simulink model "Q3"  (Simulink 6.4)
settings: Solver=ode4  StartTime=0.0  StopTime=10  FixedStep=0.01  RelTol=1e-3
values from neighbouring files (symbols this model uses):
  A = pi*R^2    (= 0.0669661890039)    [par.m]
  a = 14    [par.m]
  Cd = 0.02    [par.m]
  Cd_sfe = 0.24    [par.m]
  g = 9.81    [par.m]
  h = -0.012    [par.m]
  I = diag([Ix Iy Iz])    [par.m]
  I_inv = inv(I)    [par.m]
  J = Ja+Jr/(n^2)    (= 2.07047193878e-06)    [par.m]
  Ja = 1e-006    (= 1e-06)    [par.m]
  Jr = 3.357e-005    (= 3.357e-05)    [par.m]
  K = 0.00345    [par.m]
  l = 0.237    [par.m]
  m = 0.488    [par.m]
  Minv = inv(M)    [par.m]
  n = 5.6    [par.m]
  omegah = x    (= 300)    [par.m]
  r = 0.1    [par.m]
  R = 0.146    [par.m]
  rho = 1.225    [par.m]
  s = b*c*R/A    (= 0.100289416195)    [par.m]
  tau = Ra*J/K^2    (= 0.22300735354)    [par.m]
  teta = 0.22    [par.m]
  x0 = []    [betaDx.m]    (also in alfa.m; control.m = zeros(16,1); beta.m; lambda.m)
libraries: aerolibutil x11, simulink x8, aerosimlib x8
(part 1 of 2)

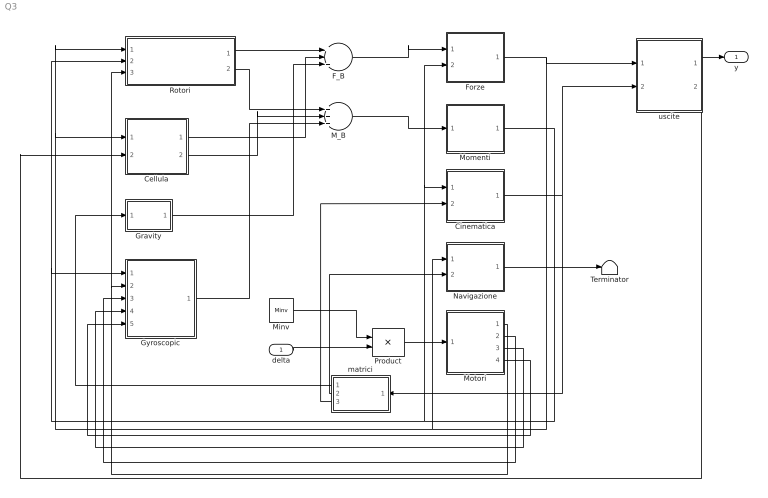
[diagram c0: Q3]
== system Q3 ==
  delta : Inport
  Cellula : Subsystem
  Cinematica : Subsystem
  F_B : Sum  Inputs=+++  OutScaling=2^-10
  Forze : Subsystem
  Gravity : Subsystem
  Gyroscopic : Subsystem
  M_B : Sum  Inputs=+++  OutScaling=2^-10
  Minv : Constant  Value=Minv  OutDataType=sfix(16)  ConRadixGroup=Use specified scaling  OutScaling=2^0  SampleTime=inf  FramePeriod=inf
  Momenti : Subsystem
  Motori : Subsystem
  Navigazione : Subsystem
  Product : Product  Multiplication=Matrix(*)
  Rotori : Subsystem
  Terminator : Terminator
  matrici : Subsystem  Orientation=left
  uscite : Subsystem
  y : Outport
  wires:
  Rotori/1(F_R) -> F_B/1
  Cellula/1(F_C) -> F_B/2
  Rotori/2(M_R) -> M_B/1
  Cellula/2(M_C) -> M_B/2
  F_B/1 -> Forze/1(F_B)
  M_B/1 -> Momenti/1(M_B)
  Cinematica/1(Euler) -> matrici/1(Euler), uscite/2(Euler)
  matrici/3(R_inv) -> Cinematica/2(R_inv)
  Momenti/1(omegaB) -> Gyroscopic/1(omegaB), Rotori/2(omegaB), Cinematica/1(omegaB), Forze/2(omegaB)
  Forze/1(velB) -> Cellula/1(velB), Rotori/1(velB), Navigazione/1(velB), uscite/1(velB)
  Motori/1(omega_r) -> Gyroscopic/2(omega_r), Rotori/3(omega_r)
  Product/1 -> Motori/1(Va)
  Motori/2(omega_m) -> Gyroscopic/3(omega_m)
  Motori/3(omega_r_dot) -> Gyroscopic/4(omega_r_dot)
  Motori/4(omega_m_dot) -> Gyroscopic/5(omega_m_dot)
  matrici/1(L_BE) -> Gravity/1(L_BE)
  matrici/2(L_EB) -> Navigazione/2(L_EB)
  uscite/1(y) -> y/1
  Navigazione/1(NED) -> Terminator/1
  uscite/2(ab) -> Cellula/2(ab)
  Minv/1 -> Product/1
  delta/1 -> Product/2
  Gyroscopic/1(M_G) -> M_B/3
  Gravity/1(F_g) -> F_B/3

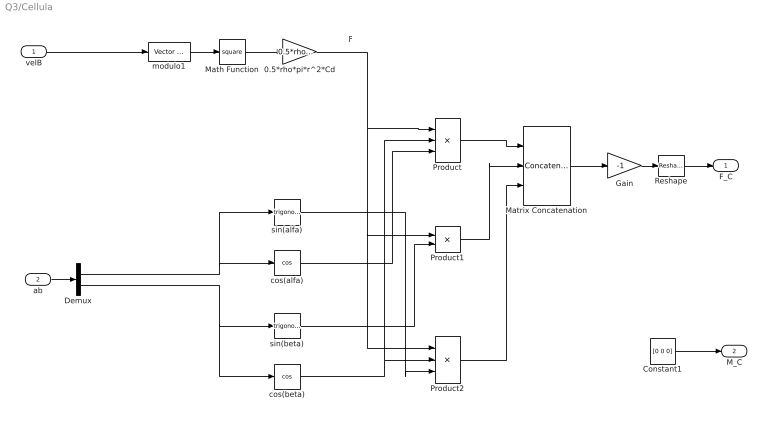
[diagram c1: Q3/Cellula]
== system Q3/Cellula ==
  note: F
  velB : Inport
  ab : Inport  Port=2
  0.5*rho*pi*r^2*Cd : Gain  Gain=0.5*rho*pi*r^2*Cd_sfe
  Constant1 : Constant  Value=[0 0 0]  OutDataType=sfix(16)  ConRadixGroup=Use specified scaling  OutScaling=2^0  SampleTime=inf  FramePeriod=inf
  Demux : Demux  Outputs=2
  Gain : Gain  Gain=-1
  Math Function : Math  Operator=square
  Matrix Concatenation : Concatenate  NumInputs=3  Mode=Vertical matrix concatenation
  Product : Product  Inputs=3
  Product1 : Product
  Product2 : Product  Inputs=3
  Reshape : simulink/Math Operations/Reshape  OutputDimensionality=1-D array  OutputDimensions=[1,1]
  cos(alfa) : Trigonometry  Operator=cos
  cos(beta) : Trigonometry  Operator=cos
  modulo1 : aerosimlib/Math/Vector norm  SystemSampleTime=-1
  sin(alfa) : Trigonometry
  sin(beta) : Trigonometry
  F_C : Outport
  M_C : Outport  Port=2
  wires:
  modulo1/1 -> Math Function/1
  Math Function/1 -> 0.5*rho*pi*r^2*Cd/1
  Constant1/1 -> M_C/1
  ab/1 -> Demux/1
  Demux/1 -> cos(alfa)/1, sin(alfa)/1
  Demux/2 -> sin(beta)/1, cos(beta)/1
  0.5*rho*pi*r^2*Cd/1 -> Product/1, Product1/1, Product2/1
  cos(beta)/1 -> Product/2, Product2/2
  cos(alfa)/1 -> Product/3
  sin(beta)/1 -> Product1/2
  sin(alfa)/1 -> Product2/3
  Product/1 -> Matrix Concatenation/1
  Product1/1 -> Matrix Concatenation/2
  Product2/1 -> Matrix Concatenation/3
  Matrix Concatenation/1 -> Gain/1
  Gain/1 -> Reshape/1
  Reshape/1 -> F_C/1
  velB/1 -> modulo1/1

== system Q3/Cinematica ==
  note: [p q r]
  note: Euler_dot
  note: [phi teta psi]
  omegaB : Inport
  R_inv : Inport  Port=2
  Integrator : Integrator  InitialCondition=[x0(4) x0(5) x0(6)]
  Product : Product  Multiplication=Matrix(*)
  Euler : Outport
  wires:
  R_inv/1 -> Product/1
  omegaB/1 -> Product/2
  Product/1 -> Integrator/1
  Integrator/1 -> Euler/1

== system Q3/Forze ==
  note: [X Y Z]
  note: acc
  note: vel_dot
  note: [u v w]
  F_B : Inport
  omegaB : Inport  Port=2
  Divide : Product  Inputs=*/  OutScaling=2^-10
  Gain : Gain  Gain=-1
  Integrator : Integrator  InitialCondition=[x0(1) x0(2) x0(3)]
  Sum : Sum  Inputs=++|
  massa : Constant  Value=m  OutDataType=sfix(16)  ConRadixGroup=Use specified scaling  OutScaling=2^0  SampleTime=inf  FramePeriod=inf
  omegaB x vel : aerolibutil/3x3 Cross Product  SystemSampleTime=-1
  velB : Outport
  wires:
  omegaB/1 -> omegaB x vel/1
  omegaB x vel/1 -> Gain/1
  F_B/1 -> Divide/1
  massa/1 -> Divide/2
  Divide/1 -> Sum/1
  Gain/1 -> Sum/2
  Sum/1 -> Integrator/1
  Integrator/1 -> velB/1, omegaB x vel/2

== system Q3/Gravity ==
  L_BE : Inport
  Constant : Constant  Value=[0 0 m*g]'  OutDataType=sfix(16)  ConRadixGroup=Use specified scaling  OutScaling=2^0  SampleTime=inf  FramePeriod=inf
  L_BE1 : Product  Multiplication=Matrix(*)
  F_g : Outport
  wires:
  Constant/1 -> L_BE1/2
  L_BE1/1 -> F_g/1
  L_BE/1 -> L_BE1/1

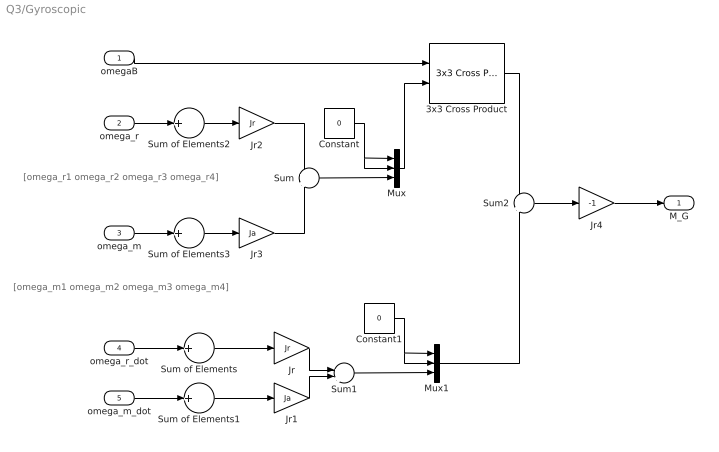
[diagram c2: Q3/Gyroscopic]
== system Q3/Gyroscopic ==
  note: [omega_r1 omega_r2 omega_r3 omega_r4]
  note: [omega_m1 omega_m2 omega_m3 omega_m4]
  omegaB : Inport
  omega_r : Inport  Port=2
  omega_m : Inport  Port=3
  omega_r_dot : Inport  Port=4
  omega_m_dot : Inport  Port=5
  3x3 Cross Product : aerolibutil/3x3 Cross Product  SystemSampleTime=-1
  Constant : Constant  Value=0  OutDataType=sfix(16)  ConRadixGroup=Use specified scaling  OutScaling=2^0  SampleTime=inf  FramePeriod=inf
  Constant1 : Constant  Value=0  OutDataType=sfix(16)  ConRadixGroup=Use specified scaling  OutScaling=2^0  SampleTime=inf  FramePeriod=inf
  Jr : Gain  Gain=Jr
  Jr1 : Gain  Gain=Ja
  Jr2 : Gain  Gain=Jr
  Jr3 : Gain  Gain=Ja
  Jr4 : Gain  Gain=-1
  Mux : Mux  Inputs=3
  Mux1 : Mux  Inputs=3
  Sum : Sum  Inputs=+|+
  Sum of Elements{,1..3} (4 alike) : Sum  Inputs=+  OutScaling=2^-10
  Sum1 : Sum  Inputs=+|+
  Sum2 : Sum  Inputs=+|+
  M_G : Outport
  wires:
  omega_r_dot/1 -> Sum of Elements/1
  omega_m_dot/1 -> Sum of Elements1/1
  Sum of Elements/1 -> Jr/1
  Sum of Elements1/1 -> Jr1/1
  omegaB/1 -> 3x3 Cross Product/1
  omega_r/1 -> Sum of Elements2/1
  omega_m/1 -> Sum of Elements3/1
  Sum of Elements2/1 -> Jr2/1
  Sum of Elements3/1 -> Jr3/1
  Jr2/1 -> Sum/1
  Jr3/1 -> Sum/2
  Jr/1 -> Sum1/1
  Jr1/1 -> Sum1/2
  Sum2/1 -> Jr4/1
  Jr4/1 -> M_G/1
  Sum/1 -> Mux/3
  Constant/1 -> Mux/1, Mux/2
  Mux/1 -> 3x3 Cross Product/2
  3x3 Cross Product/1 -> Sum2/1
  Sum1/1 -> Mux1/3
  Constant1/1 -> Mux1/1, Mux1/2
  Mux1/1 -> Sum2/2

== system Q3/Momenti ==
  note: [l m n]
  note: omegaB_dot
  M_B : Inport
  Gain : Gain  Gain=-1
  I * omegaB : Product  Multiplication=Matrix(*)
  I*omegaB2 : Product  Multiplication=Matrix(*)
  Integrator : Integrator  InitialCondition=[x0(7) x0(8) x0(9)]
  Scope3 : Scope
  Sum : Sum  Inputs=|++
  matrice d'inerzia  inversa in assi corpo : Constant  Value=I_inv  OutDataType=sfix(16)  ConRadixGroup=Use specified scaling  OutScaling=2^0  SampleTime=inf  FramePeriod=inf
  matrice d'inerzia in assi corpo : Constant  Value=I  OutDataType=sfix(16)  ConRadixGroup=Use specified scaling  OutScaling=2^0  SampleTime=inf  FramePeriod=inf
  omegaB x (I * omegaB) : aerolibutil/3x3 Cross Product  SystemSampleTime=-1
  omegaB : Outport
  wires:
  matrice d'inerzia in assi corpo/1 -> I * omegaB/1
  I * omegaB/1 -> omegaB x (I * omegaB)/2
  omegaB x (I * omegaB)/1 -> Gain/1
  Gain/1 -> Sum/1
  M_B/1 -> Sum/2
  Integrator/1 -> omegaB/1, I * omegaB/2, omegaB x (I * omegaB)/1
  matrice d'inerzia  inversa in assi corpo/1 -> I*omegaB2/1
  Sum/1 -> I*omegaB2/2
  I*omegaB2/1 -> Integrator/1, Scope3/1

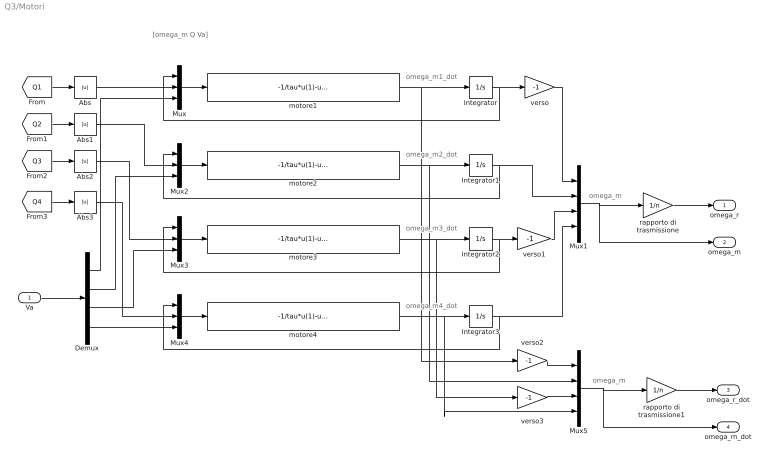
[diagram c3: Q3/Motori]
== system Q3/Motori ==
  note: [omega_m Q Va]
  note: omega_m1_dot
  note: omega_m2_dot
  note: omega_m3_dot
  note: omega_m4_dot
  note: omega_m
  note: omega_m
  Va : Inport
  Abs{,1..3} (4 alike) : Abs  SampleTime=-1
  Demux : Demux
  Integrator : Integrator  InitialCondition=x0(10)
  Integrator1 : Integrator  InitialCondition=x0(11)
  Integrator2 : Integrator  InitialCondition=x0(12)
  Integrator3 : Integrator  InitialCondition=x0(13)
  Mux{,2..4} (4 alike) : Mux  Inputs=3
  Mux1 : Mux
  Mux5 : Mux
  motore{1..4} (4 alike) : Fcn  Expr=-1/tau*u(1)-u(2)/J/n+1/K/tau*u(3)
  rapporto di trasmissione : Gain  Gain=1/n
  rapporto di trasmissione1 : Gain  Gain=1/n
  verso{,1..3} (4 alike) : Gain  Gain=-1
  omega_r : Outport
  omega_m : Outport  Port=2
  omega_r_dot : Outport  Port=3
  omega_m_dot : Outport  Port=4
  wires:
  Mux/1 -> motore1/1
  motore1/1 -> Integrator/1, verso2/1
  Integrator/1 -> Mux/1, verso/1
  Mux1/1 -> rapporto di trasmissione/1, omega_m/1
  Va/1 -> Demux/1
  Demux/1 -> Mux/3
  Mux2/1 -> motore2/1
  motore2/1 -> Integrator1/1, Mux5/2
  Integrator1/1 -> Mux2/1, Mux1/2
  Mux3/1 -> motore3/1
  motore3/1 -> Integrator2/1, verso3/1
  Integrator2/1 -> Mux3/1, verso1/1
  Mux4/1 -> motore4/1
  motore4/1 -> Integrator3/1, Mux5/4
  Integrator3/1 -> Mux4/1, Mux1/4
  Demux/2 -> Mux2/3
  Demux/3 -> Mux3/3
  Demux/4 -> Mux4/3
  [Q1] -> Abs/1
  [Q2] -> Abs1/1
  [Q3] -> Abs2/1
  [Q4] -> Abs3/1
  rapporto di trasmissione/1 -> omega_r/1
  Mux5/1 -> omega_m_dot/1, rapporto di trasmissione1/1
  rapporto di trasmissione1/1 -> omega_r_dot/1
  Abs/1 -> Mux/2
  Abs1/1 -> Mux2/2
  Abs2/1 -> Mux3/2
  Abs3/1 -> Mux4/2
  verso3/1 -> Mux5/3
  verso2/1 -> Mux5/1
  verso1/1 -> Mux1/3
  verso/1 -> Mux1/1

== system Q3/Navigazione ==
  note: [u v w]
  note: NED_dot
  note: [N E D]
  velB : Inport
  L_EB : Inport  Port=2
  Integrator : Integrator  InitialCondition=[x0(14) x0(15) x0(16)]
  Product : Product  Multiplication=Matrix(*)
  NED : Outport
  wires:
  velB/1 -> Product/2
  Product/1 -> Integrator/1
  Integrator/1 -> NED/1
  L_EB/1 -> Product/1

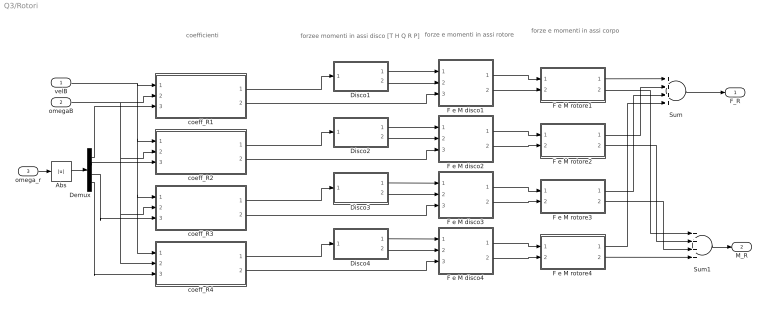
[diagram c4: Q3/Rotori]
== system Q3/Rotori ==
  note: coefficienti
  note: forzee momenti in assi disco [T H Q R P]
  note: forze e momenti in assi rotore
  note: forze e momenti in assi corpo
  velB : Inport
  omegaB : Inport  Port=2
  omega_r : Inport  Port=3
  Abs : Abs  SampleTime=-1
  Demux : Demux
  Disco1 : Subsystem
  Disco2 : Subsystem
  Disco3 : Subsystem
  Disco4 : Subsystem
  F e M disco1 : Subsystem
  F e M disco2 : Subsystem
  F e M disco3 : Subsystem
  F e M disco4 : Subsystem
  F e M rotore1 : Subsystem
  F e M rotore2 : Subsystem
  F e M rotore3 : Subsystem
  F e M rotore4 : Subsystem
  Sum : Sum  Inputs=++++
  Sum1 : Sum  Inputs=++++
  coeff_R1 : Subsystem
  coeff_R2 : Subsystem
  coeff_R3 : Subsystem
  coeff_R4 : Subsystem
  F_R : Outport
  M_R : Outport  Port=2
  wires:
  F e M disco1/1(F_disco1) -> F e M rotore1/1(F_disco1)
  F e M disco1/2(M_disco1) -> F e M rotore1/2(M_disco1)
  F e M disco2/1(F_disco2) -> F e M rotore2/1(F_disco2)
  F e M disco2/2(M_disco2) -> F e M rotore2/2(M_disco2)
  F e M disco3/1(F_disco3) -> F e M rotore3/1(F_disco3)
  F e M disco3/2(M_disco3) -> F e M rotore3/2(M_disco3)
  F e M disco4/1(F_disco4) -> F e M rotore4/1(F_disco4)
  F e M disco4/2(M_disco4) -> F e M rotore4/2(M_disco4)
  Disco1/1(F_D1) -> F e M disco1/1(F_D1)
  Disco1/2(M_D1) -> F e M disco1/2(M_D1)
  Disco2/1(F_D2) -> F e M disco2/1(F_D2)
  Disco2/2(M_D2) -> F e M disco2/2(M_D2)
  Disco3/1(F_D3) -> F e M disco3/1(F_D3)
  Disco3/2(M_D3) -> F e M disco3/2(M_D3)
  Disco4/1(F_D4) -> F e M disco4/1(F_D4)
  Disco4/2(M_D4) -> F e M disco4/2(M_D4)
  coeff_R4/1(coeff4) -> Disco4/1(coeff4)
  coeff_R3/1(coeff3) -> Disco3/1(coeff3)
  coeff_R2/1(coeff2) -> Disco2/1(coeff2)
  coeff_R1/1(coeff1) -> Disco1/1(coeff1)
  coeff_R1/2(L_RD1) -> F e M disco1/3(L_RD1)
  coeff_R2/2(L_RD2) -> F e M disco2/3(L_RD2)
  coeff_R3/2(L_RD3) -> F e M disco3/3(L_RD3)
  coeff_R4/2(L_RD4) -> F e M disco4/3(L_RD4)
  velB/1 -> coeff_R4/1(velB), coeff_R3/1(velB), coeff_R2/1(velB), coeff_R1/1(velB)
  omegaB/1 -> coeff_R3/2(omegaB), coeff_R4/2(omegaB), coeff_R2/2(omegaB), coeff_R1/2(omegaB)
  F e M rotore1/1(F_R1) -> Sum/1
  F e M rotore2/1(F_R2) -> Sum/2
  F e M rotore3/1(F_R3) -> Sum/3
  F e M rotore4/1(F_R4) -> Sum/4
  Sum/1 -> F_R/1
  F e M rotore1/2(M_R1) -> Sum1/1
  F e M rotore2/2(M_R2) -> Sum1/2
  F e M rotore3/2(M_R3) -> Sum1/3
  F e M rotore4/2(M_R4) -> Sum1/4
  Sum1/1 -> M_R/1
  omega_r/1 -> Abs/1
  Demux/1 -> coeff_R1/3(omega_r1)
  Demux/2 -> coeff_R2/3(omega_r2)
  Demux/3 -> coeff_R3/3(omega_r3)
  Demux/4 -> coeff_R4/3(omega_r4)
  Abs/1 -> Demux/1

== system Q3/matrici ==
  Euler : Inport
  Subsystem1 : Subsystem
  Subsystem2 : Subsystem
  hlpfcn : Subsystem
  L_BE : Outport
  L_EB : Outport  Port=2
  R_inv : Outport  Port=3
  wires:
  hlpfcn/1(hlpfcn) -> Subsystem1/1(hlpfcn), Subsystem2/1(hlpfcn)
  Subsystem1/1(L_BE) -> L_BE/1
  Euler/1 -> hlpfcn/1(Euler)
  Subsystem2/1(R_inv) -> R_inv/1
  Subsystem1/2(L_EB) -> L_EB/1

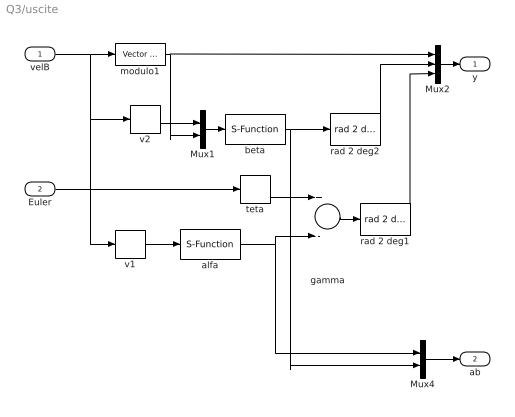
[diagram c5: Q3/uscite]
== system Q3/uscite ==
  velB : Inport
  Euler : Inport  Port=2
  Mux1 : Mux  Inputs=2
  Mux2 : Mux  Inputs=3
  Mux4 : Mux  Inputs=2
  alfa : S-Function  FunctionName=alfa
  beta : S-Function  FunctionName=beta
  gamma : Sum  Inputs=+-  OutScaling=2^-10
  modulo1 : aerosimlib/Math/Vector norm  SystemSampleTime=-1
  rad 2 deg1 : aerosimlib/Unit Conversion/Angular position/rad 2 deg  SystemSampleTime=-1
  rad 2 deg2 : aerosimlib/Unit Conversion/Angular position/rad 2 deg  SystemSampleTime=-1
  teta : Selector  Elements=2  InputPortWidth=3
  v1 : Selector  Elements=[1 3]  InputPortWidth=3
  v2 : Selector  Elements=2  InputPortWidth=3
  y : Outport
  ab : Outport  Port=2
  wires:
  modulo1/1 -> Mux1/2, Mux2/1
  Mux1/1 -> beta/1
  v2/1 -> Mux1/1
  beta/1 -> rad 2 deg2/1, Mux4/2
  rad 2 deg2/1 -> Mux2/2
  Mux2/1 -> y/1
  teta/1 -> gamma/1
  gamma/1 -> rad 2 deg1/1
  alfa/1 -> gamma/2, Mux4/1
  v1/1 -> alfa/1
  rad 2 deg1/1 -> Mux2/3
  Euler/1 -> teta/1
  velB/1 -> modulo1/1, v2/1, v1/1
  Mux4/1 -> ab/1

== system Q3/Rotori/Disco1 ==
  coeff1 : Inport
  Constant : Constant  Value=0  OutDataType=sfix(16)  ConRadixGroup=Use specified scaling  OutScaling=2^0  SampleTime=inf  FramePeriod=inf
  H : Fcn  Expr=-rho*s*A*u(1)^2*R^2*u(3)
  Mux : Mux  Inputs=3
  Mux1 : Mux  Inputs=3
  Mux2 : Mux  Inputs=[1 5]
  P : Fcn  Expr=rho*s*A*u(1)^2*R^3*u(6)
  Q : Fcn  Expr=rho*s*A*u(1)^2*R^3*u(4)
  R : Fcn  Expr=-rho*s*A*u(1)^2*R^3*u(5)
  T : Fcn  Expr=-rho*s*A*u(1)^2*R^2*u(2)
  omegah : Constant  Value=omegah  OutDataType=sfix(16)  ConRadixGroup=Use specified scaling  OutScaling=2^0  SampleTime=inf  FramePeriod=inf
  F_D1 : Outport
  M_D1 : Outport  Port=2
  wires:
  Constant/1 -> Mux/2
  H/1 -> Mux/1
  T/1 -> Mux/3
  R/1 -> Mux1/1
  Q/1 -> Mux1/3, [Q1]
  Mux/1 -> F_D1/1
  Mux1/1 -> M_D1/1
  Mux2/1 -> T/1, Q/1, R/1, P/1, H/1
  omegah/1 -> Mux2/1
  coeff1/1 -> Mux2/2
  P/1 -> Mux1/2

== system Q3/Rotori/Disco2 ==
  coeff2 : Inport
  Constant : Constant  Value=0  OutDataType=sfix(16)  ConRadixGroup=Use specified scaling  OutScaling=2^0  SampleTime=inf  FramePeriod=inf
  H : Fcn  Expr=-rho*s*A*u(1)^2*R^2*u(3)
  Mux : Mux  Inputs=3
  Mux1 : Mux  Inputs=3
  Mux2 : Mux  Inputs=[1 5]
  P : Fcn  Expr=rho*s*A*u(1)^2*R^3*u(6)
  Q : Fcn  Expr=-rho*s*A*u(1)^2*R^3*u(4)
  R : Fcn  Expr=rho*s*A*u(1)^2*R^3*u(5)
  T : Fcn  Expr=-rho*s*A*u(1)^2*R^2*u(2)
  omegah : Constant  Value=omegah  OutDataType=sfix(16)  ConRadixGroup=Use specified scaling  OutScaling=2^0  SampleTime=inf  FramePeriod=inf
  F_D2 : Outport
  M_D2 : Outport  Port=2
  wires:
  Constant/1 -> Mux/2
  H/1 -> Mux/1
  T/1 -> Mux/3
  R/1 -> Mux1/1
  Q/1 -> Mux1/3, [Q2]
  Mux/1 -> F_D2/1
  Mux1/1 -> M_D2/1
  Mux2/1 -> T/1, Q/1, R/1, P/1, H/1
  omegah/1 -> Mux2/1
  coeff2/1 -> Mux2/2
  P/1 -> Mux1/2

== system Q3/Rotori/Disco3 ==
  coeff3 : Inport
  Constant : Constant  Value=0  OutDataType=sfix(16)  ConRadixGroup=Use specified scaling  OutScaling=2^0  SampleTime=inf  FramePeriod=inf
  H : Fcn  Expr=-rho*s*A*u(1)^2*R^2*u(3)
  Mux : Mux  Inputs=3
  Mux1 : Mux  Inputs=3
  Mux2 : Mux  Inputs=[1 5]
  P : Fcn  Expr=rho*s*A*u(1)^2*R^3*u(6)
  Q : Fcn  Expr=rho*s*A*u(1)^2*R^3*u(4)
  R : Fcn  Expr=-rho*s*A*u(1)^2*R^3*u(5)
  T : Fcn  Expr=-rho*s*A*u(1)^2*R^2*u(2)
  omegah : Constant  Value=omegah  OutDataType=sfix(16)  ConRadixGroup=Use specified scaling  OutScaling=2^0  SampleTime=inf  FramePeriod=inf
  F_D3 : Outport
  M_D3 : Outport  Port=2
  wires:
  Constant/1 -> Mux/2
  H/1 -> Mux/1
  T/1 -> Mux/3
  R/1 -> Mux1/1
  Q/1 -> Mux1/3, [Q3]
  Mux/1 -> F_D3/1
  Mux1/1 -> M_D3/1
  Mux2/1 -> T/1, Q/1, R/1, P/1, H/1
  omegah/1 -> Mux2/1
  coeff3/1 -> Mux2/2
  P/1 -> Mux1/2

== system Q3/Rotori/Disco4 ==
  coeff4 : Inport
  Constant : Constant  Value=0  OutDataType=sfix(16)  ConRadixGroup=Use specified scaling  OutScaling=2^0  SampleTime=inf  FramePeriod=inf
  H : Fcn  Expr=-rho*s*A*u(1)^2*R^2*u(3)
  Mux : Mux  Inputs=3
  Mux1 : Mux  Inputs=3
  Mux2 : Mux  Inputs=[1 5]
  P : Fcn  Expr=rho*s*A*u(1)^2*R^3*u(6)
  Q : Fcn  Expr=-rho*s*A*u(1)^2*R^3*u(4)
  R : Fcn  Expr=rho*s*A*u(1)^2*R^3*u(5)
  T : Fcn  Expr=-rho*s*A*u(1)^2*R^2*u(2)
  omegah : Constant  Value=omegah  OutDataType=sfix(16)  ConRadixGroup=Use specified scaling  OutScaling=2^0  SampleTime=inf  FramePeriod=inf
  F_D4 : Outport
  M_D4 : Outport  Port=2
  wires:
  Constant/1 -> Mux/2
  H/1 -> Mux/1
  T/1 -> Mux/3
  R/1 -> Mux1/1
  Q/1 -> Mux1/3, [Q4]
  Mux/1 -> F_D4/1
  Mux1/1 -> M_D4/1
  Mux2/1 -> T/1, Q/1, R/1, P/1, H/1
  omegah/1 -> Mux2/1
  coeff4/1 -> Mux2/2
  P/1 -> Mux1/2

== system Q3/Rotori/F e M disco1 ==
  note: in assi disco
  F_D1 : Inport
  M_D1 : Inport  Port=2
  L_RD1 : Inport  Port=3
  L_RD x F_D : Product  Multiplication=Matrix(*)
  Product1 : Product  Multiplication=Matrix(*)
  F_disco1 : Outport
  M_disco1 : Outport  Port=2
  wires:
  F_D1/1 -> L_RD x F_D/2
  M_D1/1 -> Product1/2
  L_RD x F_D/1 -> F_disco1/1
  Product1/1 -> M_disco1/1
  L_RD1/1 -> L_RD x F_D/1, Product1/1

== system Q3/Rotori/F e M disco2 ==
  note: in assi disco
  F_D2 : Inport
  M_D2 : Inport  Port=2
  L_RD2 : Inport  Port=3
  L_RD x F_D : Product  Multiplication=Matrix(*)
  Product1 : Product  Multiplication=Matrix(*)
  F_disco2 : Outport
  M_disco2 : Outport  Port=2
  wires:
  F_D2/1 -> L_RD x F_D/2
  M_D2/1 -> Product1/2
  L_RD x F_D/1 -> F_disco2/1
  Product1/1 -> M_disco2/1
  L_RD2/1 -> L_RD x F_D/1, Product1/1

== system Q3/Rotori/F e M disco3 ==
  note: in assi disco
  F_D3 : Inport
  M_D3 : Inport  Port=2
  L_RD3 : Inport  Port=3
  L_RD x F_D : Product  Multiplication=Matrix(*)
  Product1 : Product  Multiplication=Matrix(*)
  F_disco3 : Outport
  M_disco3 : Outport  Port=2
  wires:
  F_D3/1 -> L_RD x F_D/2
  M_D3/1 -> Product1/2
  L_RD x F_D/1 -> F_disco3/1
  Product1/1 -> M_disco3/1
  L_RD3/1 -> L_RD x F_D/1, Product1/1

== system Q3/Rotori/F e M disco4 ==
  note: in assi disco
  F_D4 : Inport
  M_D4 : Inport  Port=2
  L_RD4 : Inport  Port=3
  L_RD x F_D : Product  Multiplication=Matrix(*)
  Product1 : Product  Multiplication=Matrix(*)
  F_disco4 : Outport
  M_disco4 : Outport  Port=2
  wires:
  F_D4/1 -> L_RD x F_D/2
  M_D4/1 -> Product1/2
  L_RD x F_D/1 -> F_disco4/1
  Product1/1 -> M_disco4/1
  L_RD4/1 -> L_RD x F_D/1, Product1/1

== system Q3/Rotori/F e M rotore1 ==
  note: in assi corpo
  F_disco1 : Inport
  M_disco1 : Inport  Port=2
  Sum : Sum  Inputs=|++
  d x M_disco : aerolibutil/3x3 Cross Product  SystemSampleTime=-1
  d1 : Constant  Value=[l 0 h+t]  OutDataType=sfix(16)  ConRadixGroup=Use specified scaling  OutScaling=2^0  SampleTime=inf  FramePeriod=inf
  F_R1 : Outport
  M_R1 : Outport  Port=2
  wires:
  F_disco1/1 -> d x M_disco/2, F_R1/1
  d1/1 -> d x M_disco/1
  d x M_disco/1 -> Sum/1
  M_disco1/1 -> Sum/2
  Sum/1 -> M_R1/1

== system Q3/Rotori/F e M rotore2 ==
  note: in assi corpo
  F_disco2 : Inport
  M_disco2 : Inport  Port=2
  Sum : Sum  Inputs=|++
  d x M_disco : aerolibutil/3x3 Cross Product  SystemSampleTime=-1
  d2 : Constant  Value=[0 l h+t]  OutDataType=sfix(16)  ConRadixGroup=Use specified scaling  OutScaling=2^0  SampleTime=inf  FramePeriod=inf
  F_R2 : Outport
  M_R2 : Outport  Port=2
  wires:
  F_disco2/1 -> d x M_disco/2, F_R2/1
  d2/1 -> d x M_disco/1
  d x M_disco/1 -> Sum/1
  M_disco2/1 -> Sum/2
  Sum/1 -> M_R2/1

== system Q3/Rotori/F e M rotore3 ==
  note: in assi corpo
  F_disco3 : Inport
  M_disco3 : Inport  Port=2
  Sum : Sum  Inputs=|++
  d x M_disco : aerolibutil/3x3 Cross Product  SystemSampleTime=-1
  d3 : Constant  Value=[-l 0 h+t]  OutDataType=sfix(16)  ConRadixGroup=Use specified scaling  OutScaling=2^0  SampleTime=inf  FramePeriod=inf
  F_R3 : Outport
  M_R3 : Outport  Port=2
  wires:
  F_disco3/1 -> d x M_disco/2, F_R3/1
  d3/1 -> d x M_disco/1
  d x M_disco/1 -> Sum/1
  M_disco3/1 -> Sum/2
  Sum/1 -> M_R3/1

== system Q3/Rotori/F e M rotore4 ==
  note: in assi corpo
  F_disco4 : Inport
  M_disco4 : Inport  Port=2
  Sum : Sum  Inputs=|++
  d x M_disco : aerolibutil/3x3 Cross Product  SystemSampleTime=-1
  d4 : Constant  Value=[0 -l h+t]  OutDataType=sfix(16)  ConRadixGroup=Use specified scaling  OutScaling=2^0  SampleTime=inf  FramePeriod=inf
  F_R4 : Outport
  M_R4 : Outport  Port=2
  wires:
  F_disco4/1 -> d x M_disco/2, F_R4/1
  d4/1 -> d x M_disco/1
  d x M_disco/1 -> Sum/1
  M_disco4/1 -> Sum/2
  Sum/1 -> M_R4/1

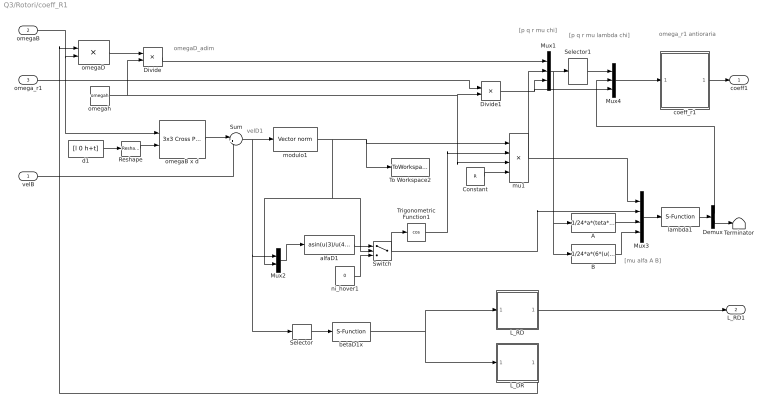
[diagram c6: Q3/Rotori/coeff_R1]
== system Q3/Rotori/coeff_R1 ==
  note: velD1
  note: omegaD_adim
  note: omega_r1 antioraria
  note: [mu alfa A B]
  note: [p q r mu chi]
  note: [p q r mu lambda chi]
  velB : Inport
  omegaB : Inport  Port=2
  omega_r1 : Inport  Port=3
  A : Fcn  Expr=1/24*a*(teta*(4*u(5)^2-8*u(5)*u(3)+4*u(3)^2+6*u(4)^2)+3*u(4)*u(1))
  B : Fcn  Expr=1/24*a*(6*(u(5)-u(3)))
  Constant : Constant  Value=R  OutDataType=sfix(16)  ConRadixGroup=Use specified scaling  OutScaling=2^0  SampleTime=inf  FramePeriod=inf
  Demux : Demux  Outputs=2
  Divide : Product  Inputs=*/  OutScaling=2^-10
  Divide1 : Product  Inputs=*/  OutScaling=2^-10
  L_DR : Subsystem
  L_RD : Subsystem
  Mux1 : Mux  Inputs=[3 1 1]
  Mux2 : Mux  Inputs=[3 1]
  Mux3 : Mux
  Mux4 : Mux  Inputs=[4 1 1]
  Reshape : simulink/Math Operations/Reshape  OutputDimensionality=Column vector  OutputDimensions=[3x1]
  Selector : Selector  Elements=[1 2]  InputPortWidth=3
  Selector1 : Selector  Elements=[1 2 3 4]  InputPortWidth=5
  Sum : Sum  Inputs=|++
  Switch : Switch  Criteria=u2 > Threshold
  Terminator : Terminator
  To Workspace2 : ToWorkspace  VariableName=Vd  SampleTime=-1  SaveFormat=Array
  Trigonometric Function1 : Trigonometry  Operator=cos
  alfaD1 : Fcn  Expr=asin(u(3)/u(4))
  betaD1x : S-Function  FunctionName=betaDx
  coeff_r1 : Subsystem
  d1 : Constant  Value=[l 0 h+t]  OutDataType=sfix(16)  ConRadixGroup=Use specified scaling  OutScaling=2^0  SampleTime=inf  FramePeriod=inf
  lambda1 : S-Function  FunctionName=lambda  Parameters=lambdah, s
  modulo1 : aerosimlib/Math/Vector norm  SystemSampleTime=-1
  mu1 : Product  Inputs=**//  OutScaling=2^-10
  ni_hover1 : Constant  Value=0  OutDataType=sfix(16)  ConRadixGroup=Use specified scaling  OutScaling=2^0  SampleTime=inf  FramePeriod=inf
  omegaB x d : aerolibutil/3x3 Cross Product  SystemSampleTime=-1
  omegaD : Product  Multiplication=Matrix(*)
  omegah : Constant  Value=omegah  OutDataType=sfix(16)  ConRadixGroup=Use specified scaling  OutScaling=2^0  SampleTime=inf  FramePeriod=inf
  coeff1 : Outport
  L_RD1 : Outport  Port=2
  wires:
  omegaB/1 -> omegaD/2, omegaB x d/1
  omegaD/1 -> Divide/1
  d1/1 -> Reshape/1
  omegaB x d/1 -> Sum/1
  velB/1 -> Sum/2
  Sum/1 -> modulo1/1, Mux2/1, Selector/1
  modulo1/1 -> Mux2/2, Switch/2, mu1/1, To Workspace2/1
  Mux2/1 -> alfaD1/1
  L_DR/1(L_DR) -> omegaD/1
  L_RD/1(L_RD1) -> L_RD1/1
  coeff_r1/1(coeff1) -> coeff1/1
  Reshape/1 -> omegaB x d/2
  omegah/1 -> Divide/2, mu1/3, Divide1/2
  Divide/1 -> Mux1/1
  Constant/1 -> mu1/4
  mu1/1 -> Mux1/2, Mux3/1
  Trigonometric Function1/1 -> mu1/2
  Mux1/1 -> A/1, B/1, Selector1/1
  Mux3/1 -> lambda1/1
  Mux4/1 -> coeff_r1/1(in_coeff)
  A/1 -> Mux3/3
  B/1 -> Mux3/4
  lambda1/1 -> Demux/1
  Demux/1 -> Mux4/2
  Demux/2 -> Terminator/1
  alfaD1/1 -> Switch/1
  ni_hover1/1 -> Switch/3
  Switch/1 -> Trigonometric Function1/1, Mux3/2
  Selector/1 -> betaD1x/1
  betaD1x/1 -> L_RD/1(betax), L_DR/1(betax)
  omega_r1/1 -> Divide1/1
  Divide1/1 -> Mux1/3, Mux4/3
  Selector1/1 -> Mux4/1

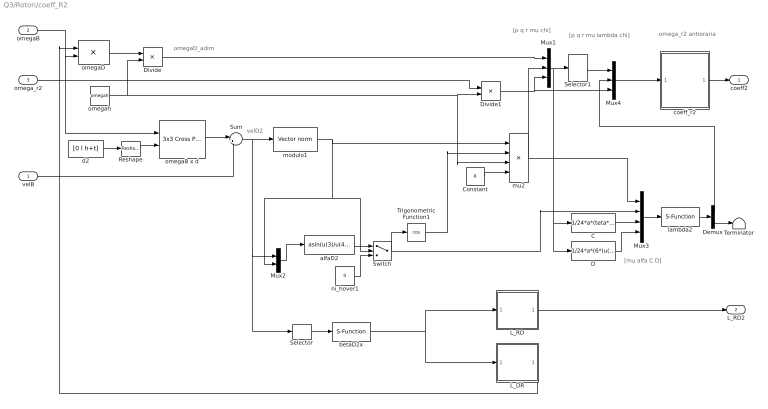
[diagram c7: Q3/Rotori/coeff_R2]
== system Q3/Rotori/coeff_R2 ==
  note: velD2
  note: omegaD_adim
  note: omega_r2 antioraria
  note: [mu alfa C D]
  note: [p q r mu chi]
  note: [p q r mu lambda chi]
  velB : Inport
  omegaB : Inport  Port=2
  omega_r2 : Inport  Port=3
  C : Fcn  Expr=1/24*a*(teta*(4*u(5)^2+8*u(5)*u(3)+4*u(3)^2+6*u(4)^2)-3*u(4)*u(1))
  Constant : Constant  Value=R  OutDataType=sfix(16)  ConRadixGroup=Use specified scaling  OutScaling=2^0  SampleTime=inf  FramePeriod=inf
  D : Fcn  Expr=1/24*a*(6*(u(5)+u(3)))
  Demux : Demux  Outputs=2
  Divide : Product  Inputs=*/  OutScaling=2^-10
  Divide1 : Product  Inputs=*/  OutScaling=2^-10
  L_DR : Subsystem
  L_RD : Subsystem
  Mux1 : Mux  Inputs=[3 1 1]
  Mux2 : Mux  Inputs=[3 1]
  Mux3 : Mux
  Mux4 : Mux  Inputs=[4 1 1]
  Reshape : simulink/Math Operations/Reshape  OutputDimensionality=Column vector  OutputDimensions=[3x1]
  Selector : Selector  Elements=[1 2]  InputPortWidth=3
  Selector1 : Selector  Elements=[1 2 3 4]  InputPortWidth=5
  Sum : Sum  Inputs=|++
  Switch : Switch  Criteria=u2 > Threshold
  Terminator : Terminator
  Trigonometric Function1 : Trigonometry  Operator=cos
  alfaD2 : Fcn  Expr=asin(u(3)/u(4))
  betaD2x : S-Function  FunctionName=betaDx
  coeff_r2 : Subsystem
  d2 : Constant  Value=[0 l h+t]  OutDataType=sfix(16)  ConRadixGroup=Use specified scaling  OutScaling=2^0  SampleTime=inf  FramePeriod=inf
  lambda2 : S-Function  FunctionName=lambda  Parameters=lambdah, s
  modulo1 : aerosimlib/Math/Vector norm  SystemSampleTime=-1
  mu2 : Product  Inputs=**//  OutScaling=2^-10
  ni_hover1 : Constant  Value=0  OutDataType=sfix(16)  ConRadixGroup=Use specified scaling  OutScaling=2^0  SampleTime=inf  FramePeriod=inf
  omegaB x d : aerolibutil/3x3 Cross Product  SystemSampleTime=-1
  omegaD : Product  Multiplication=Matrix(*)
  omegah : Constant  Value=omegah  OutDataType=sfix(16)  ConRadixGroup=Use specified scaling  OutScaling=2^0  SampleTime=inf  FramePeriod=inf
  coeff2 : Outport
  L_RD2 : Outport  Port=2
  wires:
  omegaB/1 -> omegaD/2, omegaB x d/1
  omegaD/1 -> Divide/1
  d2/1 -> Reshape/1
  omegaB x d/1 -> Sum/1
  velB/1 -> Sum/2
  Sum/1 -> Mux2/1, Selector/1, modulo1/1
  modulo1/1 -> mu2/1, Mux2/2, Switch/2
  Mux2/1 -> alfaD2/1
  L_DR/1(L_DR) -> omegaD/1
  L_RD/1(L_RD2) -> L_RD2/1
  coeff_r2/1(coeff2) -> coeff2/1
  Reshape/1 -> omegaB x d/2
  omegah/1 -> Divide/2, mu2/3, Divide1/2
  Divide/1 -> Mux1/1
  Constant/1 -> mu2/4
  mu2/1 -> Mux1/2, Mux3/1
  Trigonometric Function1/1 -> mu2/2
  Mux1/1 -> C/1, D/1, Selector1/1
  Mux3/1 -> lambda2/1
  Mux4/1 -> coeff_r2/1(in_coeff)
  C/1 -> Mux3/3
  D/1 -> Mux3/4
  lambda2/1 -> Demux/1
  Demux/1 -> Mux4/2
  Demux/2 -> Terminator/1
  alfaD2/1 -> Switch/1
  ni_hover1/1 -> Switch/3
  Switch/1 -> Trigonometric Function1/1, Mux3/2
  Selector/1 -> betaD2x/1
  betaD2x/1 -> L_RD/1(betax), L_DR/1(betax)
  omega_r2/1 -> Divide1/1
  Divide1/1 -> Mux4/3, Mux1/3
  Selector1/1 -> Mux4/1

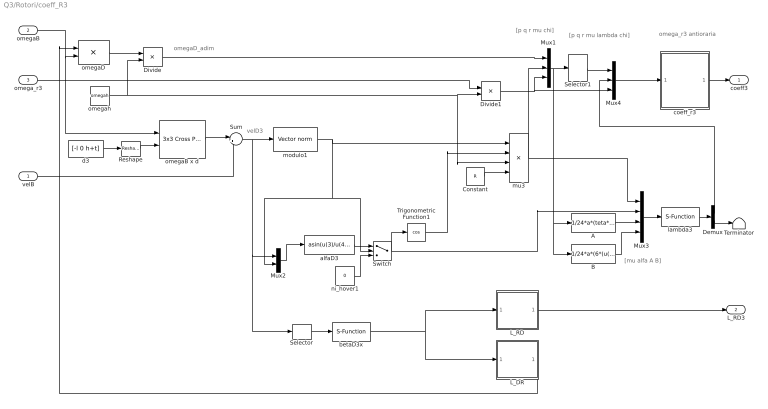
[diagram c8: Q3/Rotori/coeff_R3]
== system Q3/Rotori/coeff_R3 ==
  note: velD3
  note: omegaD_adim
  note: omega_r3 antioraria
  note: [mu alfa A B]
  note: [p q r mu chi]
  note: [p q r mu lambda chi]
  velB : Inport
  omegaB : Inport  Port=2
  omega_r3 : Inport  Port=3
  A : Fcn  Expr=1/24*a*(teta*(4*u(5)^2-8*u(5)*u(3)+4*u(3)^2+6*u(4)^2)+3*u(4)*u(1))
  B : Fcn  Expr=1/24*a*(6*(u(5)-u(3)))
  Constant : Constant  Value=R  OutDataType=sfix(16)  ConRadixGroup=Use specified scaling  OutScaling=2^0  SampleTime=inf  FramePeriod=inf
  Demux : Demux  Outputs=2
  Divide : Product  Inputs=*/  OutScaling=2^-10
  Divide1 : Product  Inputs=*/  OutScaling=2^-10
  L_DR : Subsystem
  L_RD : Subsystem
  Mux1 : Mux  Inputs=[3 1 1]
  Mux2 : Mux  Inputs=[3 1]
  Mux3 : Mux
  Mux4 : Mux  Inputs=[4 1 1]
  Reshape : simulink/Math Operations/Reshape  OutputDimensionality=Column vector  OutputDimensions=[3x1]
  Selector : Selector  Elements=[1 2]  InputPortWidth=3
  Selector1 : Selector  Elements=[1 2 3 4]  InputPortWidth=5
  Sum : Sum  Inputs=|++
  Switch : Switch  Criteria=u2 > Threshold
  Terminator : Terminator
  Trigonometric Function1 : Trigonometry  Operator=cos
  alfaD3 : Fcn  Expr=asin(u(3)/u(4))
  betaD3x : S-Function  FunctionName=betaDx
  coeff_r3 : Subsystem
  d3 : Constant  Value=[-l 0 h+t]  OutDataType=sfix(16)  ConRadixGroup=Use specified scaling  OutScaling=2^0  SampleTime=inf  FramePeriod=inf
  lambda3 : S-Function  FunctionName=lambda  Parameters=lambdah, s
  modulo1 : aerosimlib/Math/Vector norm  SystemSampleTime=-1
  mu3 : Product  Inputs=**//  OutScaling=2^-10
  ni_hover1 : Constant  Value=0  OutDataType=sfix(16)  ConRadixGroup=Use specified scaling  OutScaling=2^0  SampleTime=inf  FramePeriod=inf
  omegaB x d : aerolibutil/3x3 Cross Product  SystemSampleTime=-1
  omegaD : Product  Multiplication=Matrix(*)
  omegah : Constant  Value=omegah  OutDataType=sfix(16)  ConRadixGroup=Use specified scaling  OutScaling=2^0  SampleTime=inf  FramePeriod=inf
  coeff3 : Outport
  L_RD3 : Outport  Port=2
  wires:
  omegaB/1 -> omegaD/2, omegaB x d/1
  omegaD/1 -> Divide/1
  d3/1 -> Reshape/1
  omegaB x d/1 -> Sum/1
  velB/1 -> Sum/2
  Sum/1 -> Mux2/1, Selector/1, modulo1/1
  modulo1/1 -> mu3/1, Mux2/2, Switch/2
  Mux2/1 -> alfaD3/1
  L_DR/1(L_DR) -> omegaD/1
  L_RD/1(L_RD3) -> L_RD3/1
  coeff_r3/1(coeff3) -> coeff3/1
  Reshape/1 -> omegaB x d/2
  omegah/1 -> Divide/2, mu3/3, Divide1/2
  Divide/1 -> Mux1/1
  Constant/1 -> mu3/4
  mu3/1 -> Mux1/2, Mux3/1
  Trigonometric Function1/1 -> mu3/2
  Mux1/1 -> A/1, B/1, Selector1/1
  Mux3/1 -> lambda3/1
  Mux4/1 -> coeff_r3/1(in_coeff)
  A/1 -> Mux3/3
  B/1 -> Mux3/4
  lambda3/1 -> Demux/1
  Demux/1 -> Mux4/2
  Demux/2 -> Terminator/1
  alfaD3/1 -> Switch/1
  ni_hover1/1 -> Switch/3
  Switch/1 -> Trigonometric Function1/1, Mux3/2
  Selector/1 -> betaD3x/1
  betaD3x/1 -> L_RD/1(betax), L_DR/1(betax)
  omega_r3/1 -> Divide1/1
  Divide1/1 -> Mux4/3, Mux1/3
  Selector1/1 -> Mux4/1

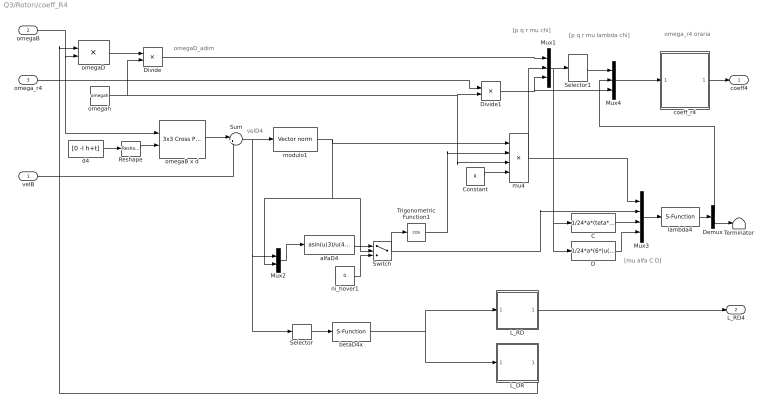
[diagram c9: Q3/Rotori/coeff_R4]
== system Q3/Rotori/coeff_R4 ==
  note: velD4
  note: omegaD_adim
  note: omega_r4 oraria
  note: [mu alfa C D]
  note: [p q r mu chi]
  note: [p q r mu lambda chi]
  velB : Inport
  omegaB : Inport  Port=2
  omega_r4 : Inport  Port=3
  C : Fcn  Expr=1/24*a*(teta*(4*u(5)^2+8*u(5)*u(3)+4*u(3)^2+6*u(4)^2)-3*u(4)*u(1))
  Constant : Constant  Value=R  OutDataType=sfix(16)  ConRadixGroup=Use specified scaling  OutScaling=2^0  SampleTime=inf  FramePeriod=inf
  D : Fcn  Expr=1/24*a*(6*(u(5)+u(3)))
  Demux : Demux  Outputs=2
  Divide : Product  Inputs=*/  OutScaling=2^-10
  Divide1 : Product  Inputs=*/  OutScaling=2^-10
  L_DR : Subsystem
  L_RD : Subsystem
  Mux1 : Mux  Inputs=[3 1 1]
  Mux2 : Mux  Inputs=[3 1]
  Mux3 : Mux
  Mux4 : Mux  Inputs=[4 1 1]
  Reshape : simulink/Math Operations/Reshape  OutputDimensionality=Column vector  OutputDimensions=[3x1]
  Selector : Selector  Elements=[1 2]  InputPortWidth=3
  Selector1 : Selector  Elements=[1 2 3 4]  InputPortWidth=5
  Sum : Sum  Inputs=|++
  Switch : Switch  Criteria=u2 > Threshold
  Terminator : Terminator
  Trigonometric Function1 : Trigonometry  Operator=cos
  alfaD4 : Fcn  Expr=asin(u(3)/u(4))
  betaD4x : S-Function  FunctionName=betaDx
  coeff_r4 : Subsystem
  d4 : Constant  Value=[0 -l h+t]  OutDataType=sfix(16)  ConRadixGroup=Use specified scaling  OutScaling=2^0  SampleTime=inf  FramePeriod=inf
  lambda4 : S-Function  FunctionName=lambda  Parameters=lambdah, s
  modulo1 : aerosimlib/Math/Vector norm  SystemSampleTime=-1
  mu4 : Product  Inputs=**//  OutScaling=2^-10
  ni_hover1 : Constant  Value=0  OutDataType=sfix(16)  ConRadixGroup=Use specified scaling  OutScaling=2^0  SampleTime=inf  FramePeriod=inf
  omegaB x d : aerolibutil/3x3 Cross Product  SystemSampleTime=-1
  omegaD : Product  Multiplication=Matrix(*)
  omegah : Constant  Value=omegah  OutDataType=sfix(16)  ConRadixGroup=Use specified scaling  OutScaling=2^0  SampleTime=inf  FramePeriod=inf
  coeff4 : Outport
  L_RD4 : Outport  Port=2
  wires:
  omegaB/1 -> omegaD/2, omegaB x d/1
  omegaD/1 -> Divide/1
  d4/1 -> Reshape/1
  omegaB x d/1 -> Sum/1
  velB/1 -> Sum/2
  Sum/1 -> Mux2/1, Selector/1, modulo1/1
  modulo1/1 -> mu4/1, Mux2/2, Switch/2
  Mux2/1 -> alfaD4/1
  L_DR/1(L_DR) -> omegaD/1
  L_RD/1(L_RD4) -> L_RD4/1
  coeff_r4/1(coeff4) -> coeff4/1
  Reshape/1 -> omegaB x d/2
  omegah/1 -> Divide/2, mu4/3, Divide1/2
  Divide/1 -> Mux1/1
  Constant/1 -> mu4/4
  mu4/1 -> Mux1/2, Mux3/1
  Trigonometric Function1/1 -> mu4/2
  Mux1/1 -> C/1, D/1, Selector1/1
  Mux3/1 -> lambda4/1
  Mux4/1 -> coeff_r4/1(in_coeff)
  C/1 -> Mux3/3
  D/1 -> Mux3/4
  lambda4/1 -> Demux/1
  Demux/1 -> Mux4/2
  Demux/2 -> Terminator/1
  alfaD4/1 -> Switch/1
  ni_hover1/1 -> Switch/3
  Switch/1 -> Trigonometric Function1/1, Mux3/2
  Selector/1 -> betaD4x/1
  betaD4x/1 -> L_RD/1(betax), L_DR/1(betax)
  omega_r4/1 -> Divide1/1
  Divide1/1 -> Mux4/3, Mux1/3
  Selector1/1 -> Mux4/1

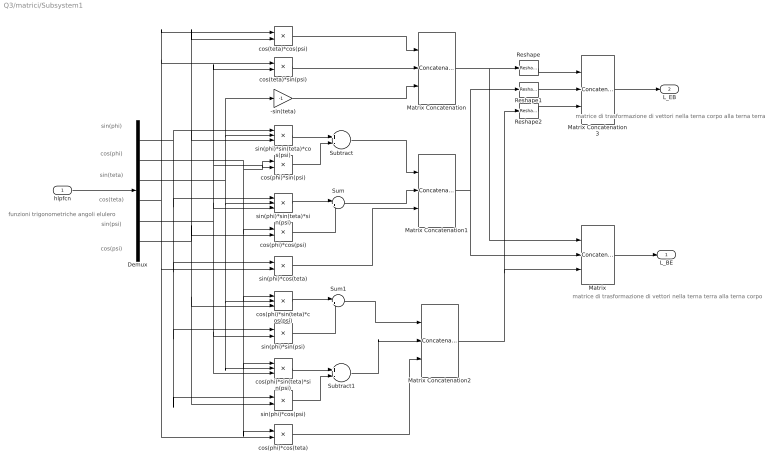
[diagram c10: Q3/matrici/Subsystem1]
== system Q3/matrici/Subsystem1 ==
  note: cos(psi)
  note: sin(psi)
  note: cos(phi)
  note: sin(phi)
  note: cos(teta)
  note: sin(teta)
  note: funzioni trigonometriche angoli elulero
  note: matrice di trasformazione di vettori nella terna terra alla terna corpo
  note: matrice di trasformazione di vettori nella terna corpo alla terna terra
  hlpfcn : Inport
  -sin(teta) : Gain  Gain=-1
  Demux : Demux  Outputs=6
  Matrix : Concatenate  NumInputs=3  Mode=Vertical matrix concatenation
  Matrix Concatenation{,1..3} (4 alike) : Concatenate  NumInputs=3  Mode=Horizontal matrix concatenation
  Reshape : simulink/Math Operations/Reshape  OutputDimensionality=Column vector  OutputDimensions=[1,1]
  Reshape1 : simulink/Math Operations/Reshape  OutputDimensionality=Column vector  OutputDimensions=[1,1]
  Reshape2 : simulink/Math Operations/Reshape  OutputDimensionality=Column vector  OutputDimensions=[1,1]
  Subtract : Sum  Inputs=+-  OutScaling=2^-10
  Subtract1 : Sum  Inputs=+-  OutScaling=2^-10
  Sum : Sum  Inputs=|++
  Sum1 : Sum  Inputs=|++
  cos(phi)*cos(psi) : Product
  cos(phi)*cos(teta) : Product
  cos(phi)*sin(psi) : Product
  cos(phi)*sin(teta)*cos(psi) : Product  Inputs=3
  cos(phi)*sin(teta)*sin(psi) : Product  Inputs=3
  cos(teta)*cos(psi) : Product
  cos(teta)*sin(psi) : Product
  sin(phi)*cos(psi) : Product
  sin(phi)*cos(teta) : Product
  sin(phi)*sin(psi) : Product
  sin(phi)*sin(teta)*cos(psi) : Product  Inputs=3
  sin(phi)*sin(teta)*sin(psi) : Product  Inputs=3
  L_BE : Outport
  L_EB : Outport  Port=2
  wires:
  Matrix/1 -> L_BE/1
  Matrix Concatenation2/1 -> Matrix/3, Reshape2/1
  Matrix Concatenation/1 -> Reshape/1, Matrix/1
  Matrix Concatenation1/1 -> Matrix/2, Reshape1/1
  cos(phi)*cos(teta)/1 -> Matrix Concatenation2/3
  Subtract1/1 -> Matrix Concatenation2/2
  sin(phi)*cos(psi)/1 -> Subtract1/2
  cos(phi)*sin(teta)*sin(psi)/1 -> Subtract1/1
  Sum1/1 -> Matrix Concatenation2/1
  sin(phi)*sin(psi)/1 -> Sum1/2
  cos(phi)*sin(teta)*cos(psi)/1 -> Sum1/1
  sin(phi)*cos(teta)/1 -> Matrix Concatenation1/3
  Sum/1 -> Matrix Concatenation1/2
  cos(phi)*cos(psi)/1 -> Sum/2
  sin(phi)*sin(teta)*sin(psi)/1 -> Sum/1
  Demux/2 -> cos(phi)*cos(teta)/1, cos(phi)*sin(teta)*sin(psi)/1, cos(phi)*sin(teta)*cos(psi)/1, cos(phi)*cos(psi)/1, cos(phi)*sin(psi)/1
  Demux/1 -> sin(phi)*cos(psi)/1, sin(phi)*sin(psi)/1, sin(phi)*cos(teta)/1, sin(phi)*sin(teta)*sin(psi)/1, sin(phi)*sin(teta)*cos(psi)/1
  Subtract/1 -> Matrix Concatenation1/1
  cos(phi)*sin(psi)/1 -> Subtract/2
  sin(phi)*sin(teta)*cos(psi)/1 -> Subtract/1
  Demux/3 -> cos(phi)*sin(teta)*sin(psi)/2, cos(phi)*sin(teta)*cos(psi)/2, sin(phi)*sin(teta)*sin(psi)/2, sin(phi)*sin(teta)*cos(psi)/2, -sin(teta)/1
  -sin(teta)/1 -> Matrix Concatenation/3
  cos(teta)*sin(psi)/1 -> Matrix Concatenation/2
  Demux/5 -> cos(phi)*sin(teta)*sin(psi)/3, sin(phi)*sin(psi)/2, sin(phi)*sin(teta)*sin(psi)/3, cos(phi)*sin(psi)/2, cos(teta)*sin(psi)/2
  cos(teta)*cos(psi)/1 -> Matrix Concatenation/1
  Demux/6 -> sin(phi)*cos(psi)/2, cos(phi)*sin(teta)*cos(psi)/3, cos(phi)*cos(psi)/2, sin(phi)*sin(teta)*cos(psi)/3, cos(teta)*cos(psi)/2
  Demux/4 -> cos(phi)*cos(teta)/2, sin(phi)*cos(teta)/2, cos(teta)*cos(psi)/1, cos(teta)*sin(psi)/1
  hlpfcn/1 -> Demux/1
  Reshape/1 -> Matrix Concatenation3/1
  Reshape1/1 -> Matrix Concatenation3/2
  Reshape2/1 -> Matrix Concatenation3/3
  Matrix Concatenation3/1 -> L_EB/1

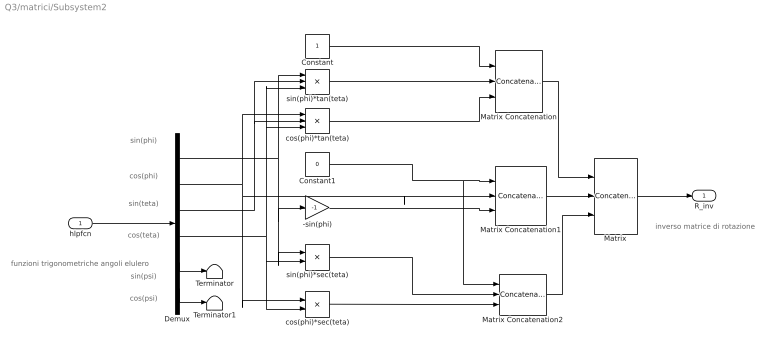
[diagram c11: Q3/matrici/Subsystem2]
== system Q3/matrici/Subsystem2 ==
  note: funzioni trigonometriche angoli elulero
  note: sin(teta)
  note: cos(teta)
  note: sin(phi)
  note: cos(phi)
  note: sin(psi)
  note: cos(psi)
  note: inverso matrice di rotazione
  hlpfcn : Inport
  -sin(phi) : Gain  Gain=-1
  Constant : Constant  Value=1  OutDataType=sfix(16)  ConRadixGroup=Use specified scaling  OutScaling=2^0  SampleTime=inf  FramePeriod=inf
  Constant1 : Constant  Value=0  OutDataType=sfix(16)  ConRadixGroup=Use specified scaling  OutScaling=2^0  SampleTime=inf  FramePeriod=inf
  Demux : Demux  Outputs=6
  Matrix : Concatenate  NumInputs=3  Mode=Vertical matrix concatenation
  Matrix Concatenation : Concatenate  NumInputs=3  Mode=Horizontal matrix concatenation
  Matrix Concatenation1 : Concatenate  NumInputs=3  Mode=Horizontal matrix concatenation
  Matrix Concatenation2 : Concatenate  NumInputs=3  Mode=Horizontal matrix concatenation
  Terminator : Terminator
  Terminator1 : Terminator
  cos(phi)*sec(teta) : Product  Inputs=*/  OutScaling=2^-10
  cos(phi)*tan(teta) : Product  Inputs=**/  OutScaling=2^-10
  sin(phi)*sec(teta) : Product  Inputs=*/  OutScaling=2^-10
  sin(phi)*tan(teta) : Product  Inputs=**/  OutScaling=2^-10
  R_inv : Outport
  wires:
  hlpfcn/1 -> Demux/1
  Demux/3 -> sin(phi)*tan(teta)/2, cos(phi)*tan(teta)/2
  Demux/1 -> sin(phi)*tan(teta)/1, -sin(phi)/1, sin(phi)*sec(teta)/1
  Demux/4 -> sin(phi)*tan(teta)/3, cos(phi)*tan(teta)/3, sin(phi)*sec(teta)/2, cos(phi)*sec(teta)/2
  Constant/1 -> Matrix Concatenation/1
  sin(phi)*tan(teta)/1 -> Matrix Concatenation/2
  Demux/2 -> cos(phi)*tan(teta)/1, Matrix Concatenation1/2, cos(phi)*sec(teta)/1
  cos(phi)*tan(teta)/1 -> Matrix Concatenation/3
  Constant1/1 -> Matrix Concatenation1/1, Matrix Concatenation2/1
  -sin(phi)/1 -> Matrix Concatenation1/3
  sin(phi)*sec(teta)/1 -> Matrix Concatenation2/2
  cos(phi)*sec(teta)/1 -> Matrix Concatenation2/3
  Demux/5 -> Terminator/1
  Demux/6 -> Terminator1/1
  Matrix/1 -> R_inv/1
  Matrix Concatenation/1 -> Matrix/1
  Matrix Concatenation1/1 -> Matrix/2
  Matrix Concatenation2/1 -> Matrix/3

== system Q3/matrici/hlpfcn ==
  note: [phi teta psi]
  Euler : Inport
  Demux : Demux  Outputs=3
  Mux : Mux  Inputs=6
  Trigonometric Function : Trigonometry
  Trigonometric Function1 : Trigonometry  Operator=cos
  Trigonometric Function2 : Trigonometry
  Trigonometric Function3 : Trigonometry  Operator=cos
  Trigonometric Function4 : Trigonometry
  Trigonometric Function5 : Trigonometry  Operator=cos
  hlpfcn : Outport
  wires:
  Euler/1 -> Demux/1
  Demux/1 -> Trigonometric Function/1, Trigonometric Function1/1
  Demux/2 -> Trigonometric Function2/1, Trigonometric Function3/1
  Demux/3 -> Trigonometric Function4/1, Trigonometric Function5/1
  Trigonometric Function/1 -> Mux/1
  Trigonometric Function1/1 -> Mux/2
  Trigonometric Function2/1 -> Mux/3
  Trigonometric Function3/1 -> Mux/4
  Trigonometric Function4/1 -> Mux/5
  Trigonometric Function5/1 -> Mux/6
  Mux/1 -> hlpfcn/1

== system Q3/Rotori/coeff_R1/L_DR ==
  betax : Inport
  Constant : Constant  Value=0  OutDataType=sfix(16)  ConRadixGroup=Use specified scaling  OutScaling=2^0  SampleTime=inf  FramePeriod=inf
  Constant1 : Constant  Value=1  OutDataType=sfix(16)  ConRadixGroup=Use specified scaling  OutScaling=2^0  SampleTime=inf  FramePeriod=inf
  Gain : Gain  Gain=-1
  Matrix Concatenation : Concatenate  NumInputs=3  Mode=Horizontal matrix concatenation
  Matrix Concatenation1 : Concatenate  NumInputs=3  Mode=Horizontal matrix concatenation
  Matrix Concatenation2 : Concatenate  NumInputs=3  Mode=Horizontal matrix concatenation
  Matrix Concatenation3 : Concatenate  NumInputs=3  Mode=Vertical matrix concatenation
  sin(beta) : Trigonometry
  sin(beta)1 : Trigonometry  Operator=cos
  L_DR : Outport
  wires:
  Matrix Concatenation3/1 -> L_DR/1
  Matrix Concatenation2/1 -> Matrix Concatenation3/3
  Matrix Concatenation1/1 -> Matrix Concatenation3/2
  Matrix Concatenation/1 -> Matrix Concatenation3/1
  Constant1/1 -> Matrix Concatenation2/3
  Constant/1 -> Matrix Concatenation2/2, Matrix Concatenation2/1, Matrix Concatenation1/3, Matrix Concatenation/3
  sin(beta)/1 -> Gain/1, Matrix Concatenation/2
  sin(beta)1/1 -> Matrix Concatenation1/2, Matrix Concatenation/1
  betax/1 -> sin(beta)/1, sin(beta)1/1
  Gain/1 -> Matrix Concatenation1/1

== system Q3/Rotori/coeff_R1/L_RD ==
  betax : Inport
  Constant : Constant  Value=0  OutDataType=sfix(16)  ConRadixGroup=Use specified scaling  OutScaling=2^0  SampleTime=inf  FramePeriod=inf
  Constant1 : Constant  Value=1  OutDataType=sfix(16)  ConRadixGroup=Use specified scaling  OutScaling=2^0  SampleTime=inf  FramePeriod=inf
  Gain : Gain  Gain=-1
  Matrix Concatenation : Concatenate  NumInputs=3  Mode=Horizontal matrix concatenation
  Matrix Concatenation1 : Concatenate  NumInputs=3  Mode=Horizontal matrix concatenation
  Matrix Concatenation2 : Concatenate  NumInputs=3  Mode=Horizontal matrix concatenation
  Matrix Concatenation3 : Concatenate  NumInputs=3  Mode=Vertical matrix concatenation
  sin(beta) : Trigonometry
  sin(beta)1 : Trigonometry  Operator=cos
  L_RD1 : Outport
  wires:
  Matrix Concatenation3/1 -> L_RD1/1
  Matrix Concatenation2/1 -> Matrix Concatenation3/3
  Matrix Concatenation1/1 -> Matrix Concatenation3/2
  Matrix Concatenation/1 -> Matrix Concatenation3/1
  Constant1/1 -> Matrix Concatenation2/3
  Constant/1 -> Matrix Concatenation2/2, Matrix Concatenation2/1, Matrix Concatenation1/3, Matrix Concatenation/3
  Gain/1 -> Matrix Concatenation/2
  sin(beta)/1 -> Matrix Concatenation1/1, Gain/1
  sin(beta)1/1 -> Matrix Concatenation1/2, Matrix Concatenation/1
  betax/1 -> sin(beta)/1, sin(beta)1/1

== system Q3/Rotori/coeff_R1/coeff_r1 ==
  note: [p_ad q_ad r_ad mu lambda chi]
  in_coeff : Inport
  Mux2 : Mux  Inputs=5
  hc : Fcn  Expr=1/4*Cd*u(4)*(u(6)-u(3))+1/12*a*(-teta*u(6)*u(1)+teta*u(3)*u(1)-3*u(5)*u(1)-3*teta*u(4)*u(5))
  pc : Fcn  Expr=1/16*a*u(2)*(u(3)-u(6))
  qc : Fcn  Expr=1/8*Cd*(u(6)^2+u(3)^2-2*u(6)*u(3)+u(4)^2)+1/48*a*(-3*u(1)^2-3*u(2)^2-4*teta*u(4)*u(1)+8*teta*u(3)*u(5)-8*teta*u(6)*u(5)-12*u(5)^2)
  rc : Fcn  Expr=-1/48*a*(u(4)*(8*teta*u(3)-8*u(6)*teta-6*u(5))+3*u(1)*(u(3)-u(6)))
  tc : Fcn  Expr=1/24*a*(teta*(4*u(6)^2-8*u(6)*u(3)+4*u(3)^2+6*u(4)^2)+6*u(5)*(u(6)-u(3))+3*u(4)*u(1))
  coeff1 : Outport
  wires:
  in_coeff/1 -> qc/1, rc/1, pc/1, hc/1, tc/1
  tc/1 -> Mux2/1
  hc/1 -> Mux2/2
  Mux2/1 -> coeff1/1
  qc/1 -> Mux2/3
  rc/1 -> Mux2/4
  pc/1 -> Mux2/5

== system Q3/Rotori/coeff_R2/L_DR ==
  betax : Inport
  Constant : Constant  Value=0  OutDataType=sfix(16)  ConRadixGroup=Use specified scaling  OutScaling=2^0  SampleTime=inf  FramePeriod=inf
  Constant1 : Constant  Value=1  OutDataType=sfix(16)  ConRadixGroup=Use specified scaling  OutScaling=2^0  SampleTime=inf  FramePeriod=inf
  Gain : Gain  Gain=-1
  Matrix Concatenation : Concatenate  NumInputs=3  Mode=Horizontal matrix concatenation
  Matrix Concatenation1 : Concatenate  NumInputs=3  Mode=Horizontal matrix concatenation
  Matrix Concatenation2 : Concatenate  NumInputs=3  Mode=Horizontal matrix concatenation
  Matrix Concatenation3 : Concatenate  NumInputs=3  Mode=Vertical matrix concatenation
  sin(beta) : Trigonometry
  sin(beta)1 : Trigonometry  Operator=cos
  L_DR : Outport
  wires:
  Matrix Concatenation3/1 -> L_DR/1
  Matrix Concatenation2/1 -> Matrix Concatenation3/3
  Matrix Concatenation1/1 -> Matrix Concatenation3/2
  Matrix Concatenation/1 -> Matrix Concatenation3/1
  Constant1/1 -> Matrix Concatenation2/3
  Constant/1 -> Matrix Concatenation2/2, Matrix Concatenation2/1, Matrix Concatenation1/3, Matrix Concatenation/3
  sin(beta)/1 -> Gain/1, Matrix Concatenation/2
  sin(beta)1/1 -> Matrix Concatenation1/2, Matrix Concatenation/1
  betax/1 -> sin(beta)/1, sin(beta)1/1
  Gain/1 -> Matrix Concatenation1/1

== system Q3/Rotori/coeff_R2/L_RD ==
  betax : Inport
  Constant : Constant  Value=0  OutDataType=sfix(16)  ConRadixGroup=Use specified scaling  OutScaling=2^0  SampleTime=inf  FramePeriod=inf
  Constant1 : Constant  Value=1  OutDataType=sfix(16)  ConRadixGroup=Use specified scaling  OutScaling=2^0  SampleTime=inf  FramePeriod=inf
  Gain : Gain  Gain=-1
  Matrix Concatenation : Concatenate  NumInputs=3  Mode=Horizontal matrix concatenation
  Matrix Concatenation1 : Concatenate  NumInputs=3  Mode=Horizontal matrix concatenation
  Matrix Concatenation2 : Concatenate  NumInputs=3  Mode=Horizontal matrix concatenation
  Matrix Concatenation3 : Concatenate  NumInputs=3  Mode=Vertical matrix concatenation
  sin(beta) : Trigonometry
  sin(beta)1 : Trigonometry  Operator=cos
  L_RD2 : Outport
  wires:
  Matrix Concatenation3/1 -> L_RD2/1
  Matrix Concatenation2/1 -> Matrix Concatenation3/3
  Matrix Concatenation1/1 -> Matrix Concatenation3/2
  Matrix Concatenation/1 -> Matrix Concatenation3/1
  Constant1/1 -> Matrix Concatenation2/3
  Constant/1 -> Matrix Concatenation2/2, Matrix Concatenation2/1, Matrix Concatenation1/3, Matrix Concatenation/3
  Gain/1 -> Matrix Concatenation/2
  sin(beta)/1 -> Matrix Concatenation1/1, Gain/1
  sin(beta)1/1 -> Matrix Concatenation1/2, Matrix Concatenation/1
  betax/1 -> sin(beta)/1, sin(beta)1/1

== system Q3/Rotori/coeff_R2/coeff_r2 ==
  note: [p_ad q_ad r_ad mu lambda chi]
  in_coeff : Inport
  Mux2 : Mux  Inputs=5
  hc : Fcn  Expr=1/4*Cd*u(4)*(u(6)+u(3))+1/12*a*(teta*u(6)*u(1)+teta*u(3)*u(1)+3*u(5)*u(1)-3*teta*u(4)*u(5))
  pc : Fcn  Expr=-1/16*a*u(2)*(u(3)+u(6))
  qc : Fcn  Expr=1/8*Cd*(u(6)^2+u(3)^2+2*u(6)*u(3)+u(4)^2)+1/48*a*(-3*u(1)^2-3*u(2)^2+4*teta*u(4)*u(1)-8*teta*u(3)*u(5)-8*teta*u(6)*u(5)-12*u(5)^2)
  rc : Fcn  Expr=-1/48*a*(u(4)*(-8*teta*u(3)-8*u(6)*teta-6*u(5))+3*u(1)*(u(3)+u(6)))
  tc : Fcn  Expr=1/24*a*(teta*(4*u(6)^2+8*u(6)*u(3)+4*u(3)^2+6*u(4)^2)+6*u(5)*(u(6)+u(3))-3*u(4)*u(1))
  coeff2 : Outport
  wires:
  in_coeff/1 -> qc/1, rc/1, pc/1, hc/1, tc/1
  tc/1 -> Mux2/1
  hc/1 -> Mux2/2
  Mux2/1 -> coeff2/1
  qc/1 -> Mux2/3
  rc/1 -> Mux2/4
  pc/1 -> Mux2/5

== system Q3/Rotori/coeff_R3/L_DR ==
  betax : Inport
  Constant : Constant  Value=0  OutDataType=sfix(16)  ConRadixGroup=Use specified scaling  OutScaling=2^0  SampleTime=inf  FramePeriod=inf
  Constant1 : Constant  Value=1  OutDataType=sfix(16)  ConRadixGroup=Use specified scaling  OutScaling=2^0  SampleTime=inf  FramePeriod=inf
  Gain : Gain  Gain=-1
  Matrix Concatenation : Concatenate  NumInputs=3  Mode=Horizontal matrix concatenation
  Matrix Concatenation1 : Concatenate  NumInputs=3  Mode=Horizontal matrix concatenation
  Matrix Concatenation2 : Concatenate  NumInputs=3  Mode=Horizontal matrix concatenation
  Matrix Concatenation3 : Concatenate  NumInputs=3  Mode=Vertical matrix concatenation
  sin(beta) : Trigonometry
  sin(beta)1 : Trigonometry  Operator=cos
  L_DR : Outport
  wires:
  Matrix Concatenation3/1 -> L_DR/1
  Matrix Concatenation2/1 -> Matrix Concatenation3/3
  Matrix Concatenation1/1 -> Matrix Concatenation3/2
  Matrix Concatenation/1 -> Matrix Concatenation3/1
  Constant1/1 -> Matrix Concatenation2/3
  Constant/1 -> Matrix Concatenation2/2, Matrix Concatenation2/1, Matrix Concatenation1/3, Matrix Concatenation/3
  sin(beta)/1 -> Gain/1, Matrix Concatenation/2
  sin(beta)1/1 -> Matrix Concatenation1/2, Matrix Concatenation/1
  betax/1 -> sin(beta)/1, sin(beta)1/1
  Gain/1 -> Matrix Concatenation1/1

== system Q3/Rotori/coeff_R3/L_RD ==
  betax : Inport
  Constant : Constant  Value=0  OutDataType=sfix(16)  ConRadixGroup=Use specified scaling  OutScaling=2^0  SampleTime=inf  FramePeriod=inf
  Constant1 : Constant  Value=1  OutDataType=sfix(16)  ConRadixGroup=Use specified scaling  OutScaling=2^0  SampleTime=inf  FramePeriod=inf
  Gain : Gain  Gain=-1
  Matrix Concatenation : Concatenate  NumInputs=3  Mode=Horizontal matrix concatenation
  Matrix Concatenation1 : Concatenate  NumInputs=3  Mode=Horizontal matrix concatenation
  Matrix Concatenation2 : Concatenate  NumInputs=3  Mode=Horizontal matrix concatenation
  Matrix Concatenation3 : Concatenate  NumInputs=3  Mode=Vertical matrix concatenation
  sin(beta) : Trigonometry
  sin(beta)1 : Trigonometry  Operator=cos
  L_RD3 : Outport
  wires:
  Matrix Concatenation3/1 -> L_RD3/1
  Matrix Concatenation2/1 -> Matrix Concatenation3/3
  Matrix Concatenation1/1 -> Matrix Concatenation3/2
  Matrix Concatenation/1 -> Matrix Concatenation3/1
  Constant1/1 -> Matrix Concatenation2/3
  Constant/1 -> Matrix Concatenation2/2, Matrix Concatenation2/1, Matrix Concatenation1/3, Matrix Concatenation/3
  Gain/1 -> Matrix Concatenation/2
  sin(beta)/1 -> Matrix Concatenation1/1, Gain/1
  sin(beta)1/1 -> Matrix Concatenation1/2, Matrix Concatenation/1
  betax/1 -> sin(beta)/1, sin(beta)1/1
